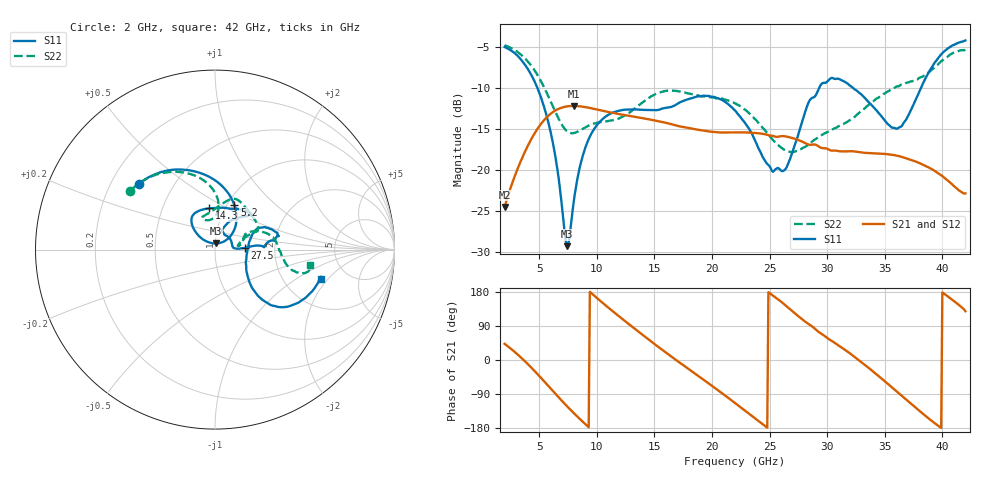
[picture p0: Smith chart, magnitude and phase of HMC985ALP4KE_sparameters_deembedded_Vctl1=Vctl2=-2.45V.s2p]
!s2p File: Measurements: S11, S21, S12, S22
# GHz S dB R 50.0
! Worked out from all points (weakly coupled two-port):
!   401 points, 2 GHz to 42 GHz, reference 50 ohm
!   highest |S21| = -12.19 dB at 8 GHz (marker M1); lowest = -24.5 dB at 2 GHz (marker M2)
!   lowest |S11| = -29.3 dB at 7.4 GHz (marker M3), VSWR 1.07, Z = 50.3 + j3.44 ohm
!   |S11| at or under -10 dB: 4.844 GHz to 29.3 GHz (24.46 GHz wide, 143 % of centre); 32.24 GHz to 38.14 GHz (5.903 GHz wide, 16.8 % of centre)
!   |S22| runs from -17.8 to -4.8 dB; largest |S21 - S12| = 0.00027
!   S11 on the Smith chart (normalised r, x): 2 GHz: 0.32, +0.34; 5.2 GHz: 1.08, +0.58; 14.3 GHz: 0.85, +0.41; 27.5 GHz: 1.40, +0.03; 42 GHz: 3.23, -1.69
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2  -5.02 139.0  -24.49 42.7  -24.49 42.7  -4.81 145.2
3.6  -6.87 105.4  -18.28 1.4  -18.28 1.4  -6.19 118.0
5.2  -11.34 66.6  -14.31 -48.6  -14.31 -48.6  -9.30 92.9
6.3  -17.50 43.1  -12.84 -85.5  -12.84 -85.5  -12.59 85.1
7.4  -29.26 82.5  -12.26 -121.4  -12.26 -121.4  -15.25 94.1
8  -23.85 135.3  -12.19 -140.0  -12.20 -140.0  -15.49 102.8
8.7  -18.68 139.8  -12.27 -160.5  -12.28 -160.5  -15.05 109.7
10.7  -13.56 128.8  -12.83 145.8  -12.84 145.8  -14.10 108.9
14.3  -12.68 98.1  -13.76 58.8  -13.77 58.8  -11.43 78.8
15.4  -12.66 84.6  -14.08 33.2  -14.09 33.2  -10.58 72.0
19.1  -10.99 45.6  -15.17 -48.3  -15.18 -48.3  -11.04 44.5
22  -12.75 51.7  -15.41 -113.3  -15.42 -113.3  -11.87 24.3
25.3  -20.20 56.0  -15.84 169.8  -15.85 169.7  -16.35 17.9
26.4  -19.86 6.6  -15.90 143.5  -15.91 143.5  -17.62 11.4
27.5  -15.63 3.2  -16.34 115.6  -16.35 115.5  -17.58 8.2
28.7  -11.21 2.8  -16.91 88.5  -16.91 88.5  -16.52 12.1
31.1  -8.96 15.4  -17.72 36.1  -17.73 36.0  -14.59 26.4
33.4  -11.43 26.3  -17.91 -15.9  -17.92 -15.9  -12.30 24.8
35.4  -14.55 6.7  -18.09 -66.4  -18.10 -66.4  -10.34 17.1
36.6  -14.35 -25.6  -18.45 -97.6  -18.46 -97.6  -9.56 10.9
39.4  -6.81 -43.5  -20.16 -168.1  -20.17 -168.2  -7.37 -13.8
42  -4.23 -15.4  -22.84 128.6  -22.84 128.6  -5.37 -9.4
